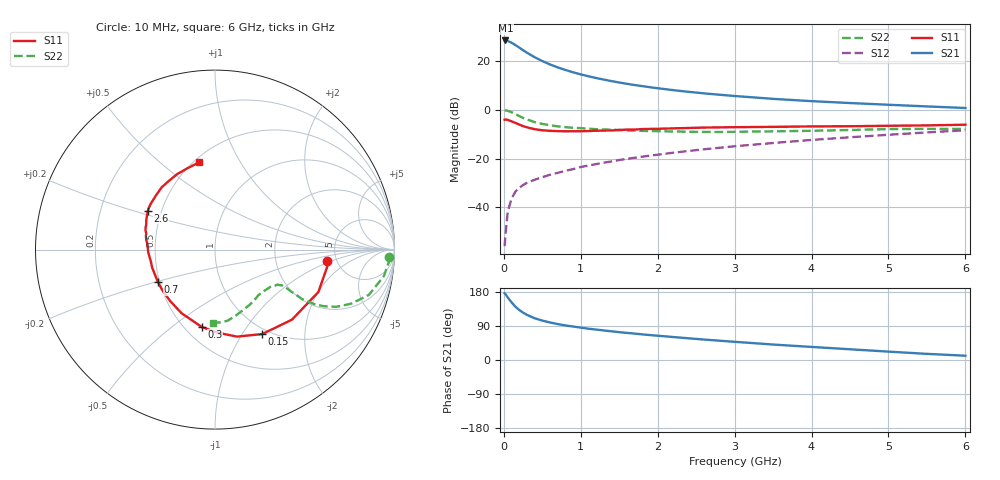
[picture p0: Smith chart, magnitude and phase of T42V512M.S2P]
! Infineon Technologies  Discrete & RF Semiconductors
! BFR182T
! Si NPN RF Bipolar Junction Transistor in SC75
! VCE = 2.5 V  IC = 12 mA
! Common Emitter S-Parameters:  October  1999
# GHz  S  MA  R  50
!  f  S11  S21  S12  S22
! GHz  MAG  ANG  MAG  ANG  MAG  ANG  MAG  ANG
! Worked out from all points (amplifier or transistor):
!   36 points, 10 MHz to 6 GHz, reference 50 ohm
!   highest |S21| = 28.4 dB at 20 MHz (marker M1)
!   |S21| within 3 dB of that: start of sweep to 203.9 MHz
!   unconditionally stable (mu >= 1): 847.8 MHz to 3.734 GHz
!   at 250 MHz: K = 0.51, MSG = 27.6 dB, |S12| = -30.8 dB
!   at 1.4 GHz: K = 1.09, MAG = 14.6 dB, |S12| = -21.2 dB
!   at 6 GHz: K = 0.84, MSG = 4.6 dB, |S12| = -8.4 dB
!   S11 on the Smith chart (normalised r, x): 10 MHz: 4.19, -0.85; 150 MHz: 0.93, -1.23; 300 MHz: 0.60, -0.65; 700 MHz: 0.49, -0.21; 2.6 GHz: 0.42, +0.22; 6 GHz: 0.53, +0.69
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0.01  0.6277 -5.6  26.43 176.0  0.0016 78.5  0.9683 -2.5
0.02  0.635 -7.6  26.44 174.2  0.0026 97.0  0.9736 -3.6
0.05  0.6225 -22.3  25.79 165.2  0.008 82.8  0.9526 -8.9
0.1  0.58 -42.3  23.72 152.2  0.0151 74.3  0.8936 -16.4
0.15  0.5391 -60.8  21.31 140.8  0.021 67.1  0.816 -21.7
0.2  0.5001 -75.8  18.9 132.0  0.0251 65.4  0.7464 -25.3
0.25  0.463 -88.3  16.7 125.0  0.0287 61.4  0.6833 -27.5
0.3  0.4376 -99.6  14.85 119.1  0.0319 60.2  0.6357 -28.7
0.4  0.4005 -117.7  12.01 110.2  0.0369 59.4  0.5598 -29.6
0.5  0.3804 -130.9  10.01 104.0  0.0415 60.0  0.5149 -29.1
0.6  0.3708 -141.8  8.51 99.0  0.0466 60.5  0.4824 -28.8
0.7  0.366 -150.1  7.421 94.9  0.051 62.5  0.4586 -28.4
0.9  0.3643 -163.8  5.878 88.3  0.0609 64.6  0.4272 -28.1
1.1  0.367 -174.0  4.876 82.6  0.0721 65.9  0.41 -28.8
1.3  0.3752 178.1  4.167 77.9  0.0824 66.8  0.3951 -30.0
1.6  0.3927 168.8  3.416 71.5  0.0988 67.4  0.3792 -32.2
2.2  0.4169 156.6  2.535 60.6  0.1318 67.6  0.36 -39.0
2.6  0.4325 149.9  2.177 54.0  0.1549 67.2  0.3525 -44.2
3.5  0.4472 136.8  1.678 40.8  0.2087 64.4  0.3623 -57.2
4.5  0.4608 124.0  1.377 28.3  0.2736 59.6  0.3857 -72.6
5.5  0.4793 108.1  1.174 16.2  0.3441 53.8  0.4069 -85.9
6  0.495 100.2  1.09 11.3  0.3812 50.0  0.4063 -91.4
